| TEXAS INSTRUMENTS INCORPORATED
| Standard Linear and Logic Group
| IBIS Model of SN74CBTLV3125
| LOW-VOLTAGE QUADRUPLE FET BUS SWITCH
| This file contains package information for the following:
|  SOIC 14-pin (D) package as [Component] CBTLV3125_D
|  TVSOP 14-pin (DGV) package as [Component] CBTLV3125_DGV
|  SOP 14-pin (NS) package as [Component] CBTLV3125_NS
|  TSSOP 14-pin (PW) package as [Component] CBTLV3125_PW
|  QSOP 16-pin (DBQ) package as [Component] CBTLV3125_DBQ
| This device can be powered at the following Vccs:
|  2.5 volt Vcc
|  3.3 volt Vcc
| This file provides unique models under the [Model Selector] for each Vcc.
| For operation at a specific Vcc, select the appropriate model after each
| [Model Selector] keyword.
[IBIS Ver]   3.2
[Comment char]  |_char
[File Name]   sn74cbtlv3125.ibs
[File Rev]   1.1 | c_die
[Date]   February 21, 2003
[Source]   Data created from TI-SPICE simulations at TI-SLL.
[Notes]   The following is an IBIS list for the CBTLV3125.
   Please contact sllibis@ti.com with questions and
   comments concerning SLL IBIS models.
   - Power-clamp data has been deleted since there is no
   power-clamp diode in the device.
   - Non-monotonic data due to device characteristics.
[Disclaimer] Property of Texas Instruments Incorporated.  Unauthorized
   reproduction and/or distribution is strictly prohibited.
   This product is protected under copyright law.
   Created  2003, (C) Copyright  2003, Texas Instruments
   Incorporated, All Rights Reserved
   UNLESS THERE IS A SIGNED, WRITTEN AGREEMENT TO THE
   CONTRARY, TEXAS INSTRUMENTS (TI) IS PROVIDING THE IBIS
   MODELS  AND WITHOUT ANY WARRANTY, EXPRESSED OR
   IMPLIED.  TI assumes no liability for:
   1) the accuracy of the IBIS models provided to your
   company;
   2) the proper functioning of these IBIS Models in your
   design or for any resulting applications; or
   3) infringement of patents, copyrights or intellectual
   property rights resulting from your use of these IBIS
   models.
   TI provides IBIS Models as a service to our customers.
   You and your company shall not distribute, sell or give
   these models to anyone else without prior written
   permission from TI.
   TI reserves the right to make changes to our products or
   to discontinue any semiconductor product or service
   without notice, and advises our customers to obtain the
   latest version of relevant information to verify, before
   placing orders, that the information being relied on is
   current.
   Please be aware that your receipt and use of the IBIS
   information provided shall serve as acceptance of these
   terms and conditions.  If you do not accept these terms,
   you should return or destroy the IBIS models and any
   other accompanying information immediately.
| Component CBTLV3125_D 14-pin SOIC
[Component]   CBTLV3125_D
[Manufacturer]   Texas Instruments, Inc.
[Package]
|   typ   min   max
R_pkg   3.100e-02   2.800e-02   3.400e-02
L_pkg   3.109e-09   2.462e-09   3.889e-09
C_pkg   4.730e-13   3.630e-13   6.280e-13
[Pin]   signal_name   model_name   R_pin   L_pin   C_pin
1   1NOE   CBTLV3125_IN   3.300e-02   3.854e-09   6.220e-13
2   1A   CBTLV3125_IO   3.200e-02   3.188e-09   4.730e-13
3   1B   CBTLV3125_IO   2.800e-02   2.462e-09   3.770e-13
4   2NOE   CBTLV3125_IN   3.100e-02   2.596e-09   3.630e-13
5   2A   CBTLV3125_IO   2.800e-02   2.521e-09   3.720e-13
6   2B   CBTLV3125_IO   3.400e-02   3.250e-09   4.760e-13
7   GND   GND   3.400e-02   3.889e-09   6.280e-13
8   3B   CBTLV3125_IO   3.400e-02   3.889e-09   6.280e-13
9   3A   CBTLV3125_IO   3.400e-02   3.250e-09   4.760e-13
10   3NOE   CBTLV3125_IN   2.800e-02   2.521e-09   3.720e-13
11   4B   CBTLV3125_IO   3.100e-02   2.596e-09   3.640e-13
12   4A   CBTLV3125_IO   2.800e-02   2.462e-09   3.770e-13
13   4NOE   CBTLV3125_IN   3.200e-02   3.188e-09   4.730e-13
14   VCC   POWER   3.300e-02   3.854e-09   6.220e-13
| Component CBTLV3125_DGV 14-pin TVSOP
[Component]   CBTLV3125_DGV
[Manufacturer]   Texas Instruments, Inc.
[Package]
|   typ   min   max
R_pkg   3.500e-02   2.000e-02   4.500e-02
L_pkg   2.499e-09   2.077e-09   2.966e-09
C_pkg   3.610e-13   3.050e-13   4.160e-13
[Pin]   signal_name   model_name   R_pin   L_pin   C_pin
1   1NOE   CBTLV3125_IN   2.700e-02   2.717e-09   3.730e-13
2   1A   CBTLV3125_IO   3.700e-02   2.434e-09   3.980e-13
3   1B   CBTLV3125_IO   3.400e-02   2.200e-09   3.160e-13
4   2NOE   CBTLV3125_IN   2.000e-02   2.077e-09   3.090e-13
5   2A   CBTLV3125_IO   3.000e-02   2.147e-09   3.050e-13
6   2B   CBTLV3125_IO   4.200e-02   2.580e-09   4.080e-13
7   GND   GND   3.900e-02   2.921e-09   3.850e-13
8   3B   CBTLV3125_IO   3.300e-02   2.841e-09   3.800e-13
9   3A   CBTLV3125_IO   4.200e-02   2.611e-09   4.100e-13
10   3NOE   CBTLV3125_IN   3.800e-02   2.331e-09   3.290e-13
11   4B   CBTLV3125_IO   2.600e-02   2.223e-09   3.190e-13
12   4A   CBTLV3125_IO   3.400e-02   2.259e-09   3.130e-13
13   4NOE   CBTLV3125_IN   4.500e-02   2.681e-09   4.160e-13
14   VCC   POWER   4.200e-02   2.966e-09   3.860e-13
| Component CBTLV3125_NS 14-pin SOP
[Component]   CBTLV3125_NS
[Manufacturer]   Texas Instruments, Inc.
[Package]
|   typ   min   max
R_pkg   4.500e-02   3.900e-02   5.400e-02
L_pkg   3.796e-09   2.561e-09   4.952e-09
C_pkg   5.280e-13   2.880e-13   7.100e-13
[Pin]   signal_name   model_name   R_pin   L_pin   C_pin
1   1NOE   CBTLV3125_IN   4.700e-02   4.867e-09   7.060e-13
2   1A   CBTLV3125_IO   5.100e-02   4.083e-09   5.920e-13
3   1B   CBTLV3125_IO   4.100e-02   2.915e-09   3.760e-13
4   2NOE   CBTLV3125_IN   3.900e-02   2.561e-09   2.880e-13
5   2A   CBTLV3125_IO   4.100e-02   3.101e-09   4.300e-13
6   2B   CBTLV3125_IO   4.700e-02   4.047e-09   5.890e-13
7   GND   GND   5.100e-02   4.909e-09   7.000e-13
8   3B   CBTLV3125_IO   4.500e-02   4.784e-09   6.940e-13
9   3A   CBTLV3125_IO   5.400e-02   4.176e-09   5.970e-13
10   3NOE   CBTLV3125_IN   3.900e-02   3.287e-09   4.490e-13
11   4B   CBTLV3125_IO   3.900e-02   2.586e-09   2.940e-13
12   4A   CBTLV3125_IO   4.000e-02   2.802e-09   3.710e-13
13   4NOE   CBTLV3125_IN   4.900e-02   4.080e-09   5.930e-13
14   VCC   POWER   5.200e-02   4.952e-09   7.100e-13
| Component CBTLV3125_PW 14-pin TSSOP
[Component]   CBTLV3125_PW
[Manufacturer]   Texas Instruments, Inc.
[Package]
|   typ   min   max
R_pkg   3.200e-02   2.900e-02   3.500e-02
L_pkg   2.378e-09   2.170e-09   2.680e-09
C_pkg   3.140e-13   2.700e-13   3.350e-13
[Pin]   signal_name   model_name   R_pin   L_pin   C_pin
1   1NOE   CBTLV3125_IN   3.300e-02   2.618e-09   3.300e-13
2   1A   CBTLV3125_IO   3.100e-02   2.313e-09   3.170e-13
3   1B   CBTLV3125_IO   3.000e-02   2.310e-09   3.140e-13
4   2NOE   CBTLV3125_IN   3.100e-02   2.173e-09   2.720e-13
5   2A   CBTLV3125_IO   3.000e-02   2.204e-09   3.090e-13
6   2B   CBTLV3125_IO   3.200e-02   2.315e-09   3.170e-13
7   GND   GND   3.500e-02   2.680e-09   3.350e-13
8   3B   CBTLV3125_IO   3.300e-02   2.640e-09   3.330e-13
9   3A   CBTLV3125_IO   3.400e-02   2.347e-09   3.190e-13
10   3NOE   CBTLV3125_IN   2.900e-02   2.277e-09   3.130e-13
11   4B   CBTLV3125_IO   3.100e-02   2.170e-09   2.700e-13
12   4A   CBTLV3125_IO   3.100e-02   2.244e-09   3.110e-13
13   4NOE   CBTLV3125_IN   3.300e-02   2.343e-09   3.210e-13
14   VCC   POWER   3.500e-02   2.657e-09   3.320e-13
| Component CBTLV3125_DBQ 16-pin QSOP
[Component]   CBTLV3125_DBQ
[Manufacturer]   Texas Instruments, Inc.
[Package]
|   typ   min   max
R_pkg   3.800e-02   2.700e-02   5.900e-02
L_pkg   2.353e-09   1.491e-09   4.500e-09
C_pkg   2.100e-13   6.400e-14   5.920e-13
[Pin]   signal_name   model_name   R_pin   L_pin   C_pin
1   NC   NC   5.800e-02   4.450e-09   5.920e-13
2   1NOE   CBTLV3125_IN   4.000e-02   1.930e-09   1.110e-13
3   1A   CBTLV3125_IO   2.800e-02   1.538e-09   7.600e-14
4   1B   CBTLV3125_IO   2.700e-02   1.491e-09   6.400e-14
5   2NOE   CBTLV3125_IN   2.700e-02   1.491e-09   6.400e-14
6   2A   CBTLV3125_IO   2.700e-02   1.506e-09   7.500e-14
7   2B   CBTLV3125_IO   3.300e-02   1.922e-09   1.090e-13
8   GND   GND   5.900e-02   4.500e-09   5.880e-13
9   NC   NC   5.800e-02   3.695e-09   4.140e-13
10   3B   CBTLV3125_IO   3.400e-02   2.685e-09   2.820e-13
11   3A   CBTLV3125_IO   2.900e-02   1.552e-09   7.700e-14
12   3NOE   CBTLV3125_IN   2.800e-02   1.506e-09   6.500e-14
13   4B   CBTLV3125_IO   2.700e-02   1.492e-09   6.400e-14
14   4A   CBTLV3125_IO   2.800e-02   1.534e-09   7.600e-14
15   4NOE   CBTLV3125_IN   4.000e-02   2.703e-09   2.840e-13
16   VCC   POWER   5.600e-02   3.645e-09   4.180e-13
[Series Switch Groups]
| Function Group States
On  1 /   | 1A->1B 1NOE LOW
On  2 /   | 2A->2B 2NOE LOW
On  3 /   | 3A->3B 3NOE LOW
On  4 /   | 4A->4B 4NOE LOW
On  1 2 3 4 /   | Enable 1 2 3 4
On  1 2 /   | Enable 1 2
On  1 3 /   | Enable 1 3
On  1 4 /   | Enable 1 4
On  2 3 /   | Enable 2 3
On  2 4 /   | Enable 2 4
On  3 4 /   | Enable 3 4
On  1 2 3 /   | Enable 1 2 3
On  1 2 4 /   | Enable 1 2 4
On  1 3 4 /   | Enable 1 3 4
On  2 3 4 /   | Enable 2 3 4
[Series Pin Mapping]   pin_2   model_name   function_table_group
2   3   CBTLV3125_IO_25_S   1
| 2   3   CBTLV3125_IO_33_S   1
5   6   CBTLV3125_IO_25_S   2
| 5   6   CBTLV3125_IO_33_S   2
9   8   CBTLV3125_IO_25_S   3
| 9   8   CBTLV3125_IO_33_S   3
12   11   CBTLV3125_IO_25_S   4
| 12   11   CBTLV3125_IO_33_S   4
| Model CBTLV3125_IN
[Model Selector]   CBTLV3125_IN
CBTLV3125_IN_25   2.5 volt Vcc
CBTLV3125_IN_33   3.3 volt Vcc
| Model CBTLV3125_IO
[Model Selector]   CBTLV3125_IO
CBTLV3125_IO_25   2.5 volt Vcc
CBTLV3125_IO_33   3.3 volt Vcc
| Model CBTLV3125_IO_S
[Model Selector]   CBTLV3125_IO_S
CBTLV3125_IO_25_S   2.5 volt Vcc
CBTLV3125_IO_33_S   3.3 volt Vcc
[Model]   CBTLV3125_IO_25_S
Model_type  Series_switch
| variable   typ   min   max
C_comp   0   0   0
[Temperature Range]   40   100   -40
| Ambient temperature   25   85   -40
[Voltage range]   2.5   2.3   2.7
[On]
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[Off]
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[Model]   CBTLV3125_IO_33_S
Model_type  Series_switch
| variable   typ   min   max
C_comp   0   0   0
[Temperature Range]   40   100   -40
| Ambient temperature   25   85   -40
[Voltage range]   3.3   3   3.6
[On]
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[Off]
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| Models and submodels in the file (6): CBTLV3125_IN_25 (Input), CBTLV3125_IN_33 (Input), CBTLV3125_IO_25_S (Series_switch), CBTLV3125_IO_25 (Terminator), CBTLV3125_IO_33_S (Series_switch), CBTLV3125_IO_33 (Terminator)
